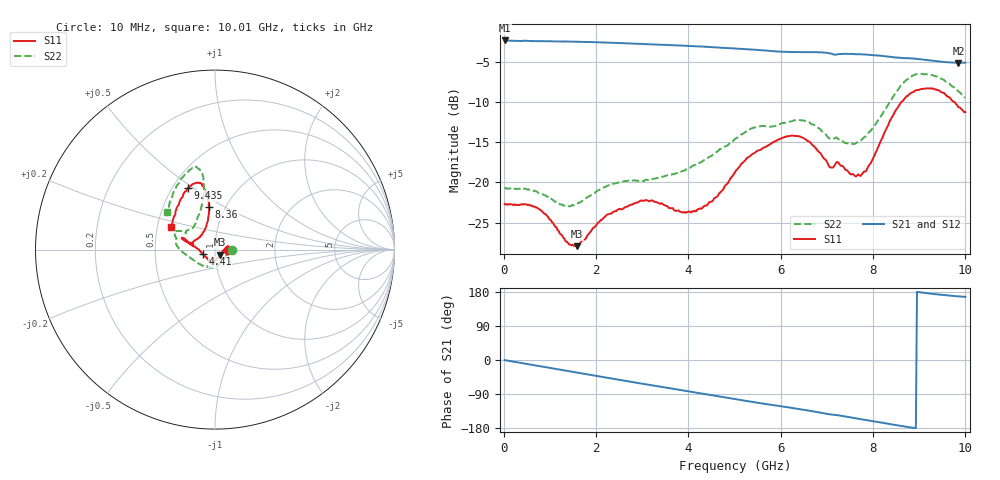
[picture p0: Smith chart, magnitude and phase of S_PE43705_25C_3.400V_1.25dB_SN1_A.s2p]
! Device ID: PE43705
! Serial: 1
! Insertion: A
! Impedance: 50 ohm
! Temp: 25C
! VDD: 3.400V
! Attenuation Step: 1.25dB
#  Hz  S  RI  R  50
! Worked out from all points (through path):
!   401 points, 10 MHz to 10.01 GHz, reference 50 ohm
!   highest |S21| = -2.28 dB at 10 MHz (marker M1); lowest = -5.1 dB at 9.86 GHz (marker M2)
!   group delay of S21, straight-line fit = 55 ps
!   lowest |S11| = -27.9 dB at 1.585 GHz (marker M3), VSWR 1.08, Z = 52.8 - j3.02 ohm
!   |S11| at or under -10 dB: start of sweep to 8.61 GHz; 9.777 GHz to end of sweep
!   |S22| runs from -23.0 to -6.4 dB; largest |S21 - S12| = 0.0068
!   S11 on the Smith chart (normalised r, x): 10 MHz: 1.16, -0.00; 4.41 GHz: 0.87, -0.04; 8.36 GHz: 0.84, +0.42; 9.435 GHz: 0.60, +0.48; 10.01 GHz: 0.59, +0.16
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1e7  0.0737 -0.000528  0.7689 -0.00404  0.7694 -0.00348  0.0928 -0.000683
7.1e8  0.0675 0.0179  0.736 -0.1967  0.7361 -0.1966  0.0877 0.00564
1.385e9  0.0393 -0.0144  0.6617 -0.3679  0.6618 -0.3677  0.0597 -0.0389
1.585e9  0.0281 -0.0285  0.6307 -0.4141  0.631 -0.4143  0.0478 -0.0562
1.685e9  0.0233 -0.0365  0.6147 -0.4362  0.6148 -0.4364  0.0401 -0.0651
2.26e9  -0.00369 -0.0632  0.5047 -0.5482  0.5051 -0.5478  0.000511 -0.0958
3.01e9  -0.0243 -0.0729  0.3329 -0.6495  0.3338 -0.6488  -0.0396 -0.0941
3.36e9  -0.0282 -0.0688  0.2497 -0.6789  0.2503 -0.6784  -0.0514 -0.0939
3.91e9  -0.0434 -0.049  0.1118 -0.7045  0.1125 -0.7045  -0.0882 -0.0794
4.41e9  -0.0686 -0.0234  -0.0134 -0.7019  -0.0127 -0.7012  -0.1331 -0.0482
5.01e9  -0.1146 0.0174  -0.1559 -0.6669  -0.1551 -0.6669  -0.1862 -0.00854
6.035e9  -0.1779 0.0647  -0.3518 -0.5514  -0.349 -0.5523  -0.2226 0.0747
6.685e9  -0.1652 0.0477  -0.4608 -0.4585  -0.4611 -0.4577  -0.2056 0.1047
7.085e9  -0.1206 0.0291  -0.5145 -0.3769  -0.5151 -0.3779  -0.1639 0.0929
7.26e9  -0.1265 0.0386  -0.5245 -0.3525  -0.5228 -0.3537  -0.1514 0.1076
7.685e9  -0.0799 0.0789  -0.5722 -0.2684  -0.5716 -0.2687  -0.1129 0.1399
7.91e9  -0.0566 0.1137  -0.5865 -0.2181  -0.5871 -0.2216  -0.0969 0.1796
8.36e9  -0.0324 0.2361  -0.5973 -0.119  -0.5954 -0.122  -0.0632 0.3094
8.835e9  -0.0689 0.3555  -0.5926 -0.02  -0.5891 -0.0208  -0.0912 0.449
9.435e9  -0.1498 0.3437  -0.564 0.0733  -0.5626 0.0732  -0.1675 0.4201
9.86e9  -0.2209 0.1954  -0.5451 0.1172  -0.545 0.116  -0.2445 0.2781
1.001e10  -0.2454 0.1239  -0.5447 0.13  -0.5472 0.1272  -0.2672 0.2086
